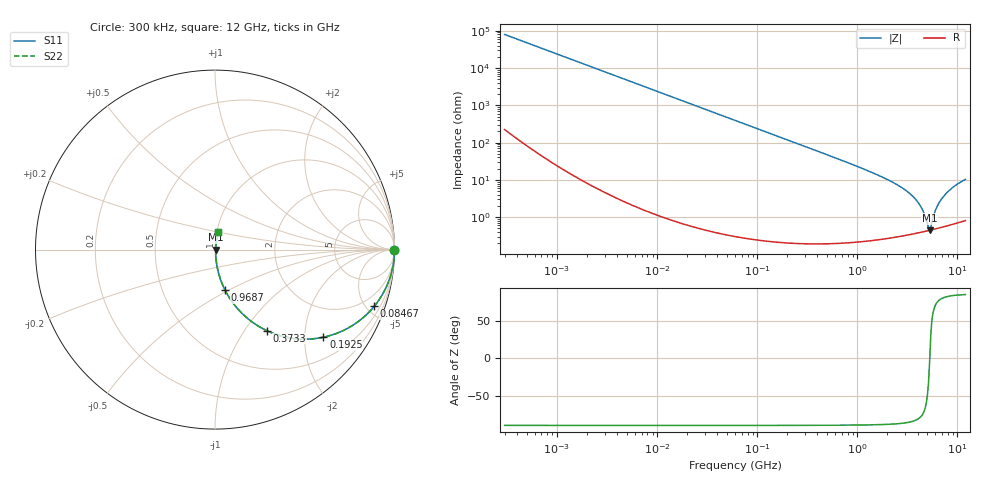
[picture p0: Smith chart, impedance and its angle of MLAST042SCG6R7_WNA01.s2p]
! MLAST042SCG6R7_WNA01  S-PARAMETER MODEL  ( General Type )
! Model Generated by TAIYO YUDEN Corporation (http://www.ty-top.com)
! Version 1.0
! TAIYO YUDEN Control No. 150820
! Copyright(c) 2015 TAIYO YUDEN CO.,LTD. All Rights Reserved.
! Product Description (link to TY-COMPAS)
! https://ds.yuden.co.jp/TYCOMPAS/or/detail?pn=MLAST042SCG6R7BWNA01&u=M
! Products Name : Multilayer Ceramic Capacitors
! Characteristics :
!  Capacitance : 6.7 pF , Rated Voltage : 25V , TCC : CG / C0G
!  Case Size : 0.4 x 0.2 / 0.016 x 0.008 [mm/inch] , Thickness : 0.2 / 0.008 [mm/inch]
!  (Conditions: Temperature = 25 degC , DC Bias Current/Voltage = 0A / 0V)
! External Node Assignments :
!  1  o---| |---o  2
! GND o---------o GND
! Frequency Range : 0.3MHz  -  12000MHz  [ 401 STEP ]
# MHz S RI R 50
! Freq[MHz].  S11 Real  S11 Imag  S21 Real  S21 Imag  S12 Real  S12 Imag  S22 Real  S22 Imag
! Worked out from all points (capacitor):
!   401 points, 300 kHz to 12 GHz, reference 50 ohm
!   read as one part in series: C = 6.68 pF near 316.3 kHz
!   lowest |Z| = 446 mohm at 5.279 GHz (marker M1)
!   series resonance near 5.29 GHz, so ESL is about 140 pH
!   S11 on the Smith chart (normalised r, x): 300 kHz: open; 84.67 MHz: 1.01, -5.62; 192.5 MHz: 1.00, -2.47; 373.3 MHz: 1.00, -1.27; 968.7 MHz: 1.00, -0.48; 12 GHz: 1.02, +0.21
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0.3  1 -0.00126  5.14e-06 0.00126  5.14e-06 0.00126  1 -0.00126
1.769972  0.9999 -0.00743  6.06e-05 0.00743  6.06e-05 0.00743  0.9999 -0.00743
10.44266  0.9981 -0.0438  0.00194 0.0438  0.00194 0.0438  0.9981 -0.0438
27.10171  0.9872 -0.1123  0.0128 0.1123  0.0128 0.1123  0.9872 -0.1123
60  0.9401 -0.2368  0.0599 0.2368  0.0599 0.2368  0.9401 -0.2368
84.66778  0.8875 -0.3155  0.1125 0.3155  0.1125 0.3155  0.8875 -0.3155
192.4766  0.6041 -0.4882  0.3959 0.4882  0.3959 0.4882  0.6041 -0.4882
353.9943  0.3102 -0.4611  0.6898 0.4611  0.6898 0.4611  0.3102 -0.4611
373.2558  0.2879 -0.4513  0.7121 0.4513  0.7121 0.4513  0.2879 -0.4513
585.5907  0.1402 -0.3447  0.8598 0.3447  0.8598 0.3447  0.1402 -0.3447
968.706  0.0553 -0.224  0.9447 0.224  0.9447 0.224  0.0553 -0.224
2088.533  0.0118 -0.0949  0.9882 0.0949  0.9882 0.0949  0.0118 -0.0949
2947.191  0.00627 -0.0553  0.9937 0.0553  0.9937 0.0553  0.00627 -0.0553
3740.715  0.00463 -0.0317  0.9954 0.0317  0.9954 0.0317  0.00463 -0.0317
4385.161  0.00425 -0.017  0.9957 0.017  0.9957 0.017  0.00425 -0.017
5006.236  0.00432 -0.0051  0.9957 0.0051  0.9957 0.0051  0.00432 -0.0051
5278.635  0.00444 -0.00024  0.9956 0.00024  0.9956 0.00024  0.00444 -0.00024
5565.855  0.00462 0.00598  0.9954 -0.00598  0.9954 -0.00598  0.00462 0.00598
6354.153  0.00542 0.0202  0.9946 -0.0202  0.9946 -0.0202  0.00542 0.0202
7254.098  0.00674 0.0353  0.9933 -0.0353  0.9933 -0.0353  0.00674 0.0353
8966.534  0.0102 0.0615  0.9898 -0.0615  0.9898 -0.0615  0.0102 0.0615
12000  0.0182 0.1001  0.9818 -0.1001  0.9818 -0.1001  0.0182 0.1001
